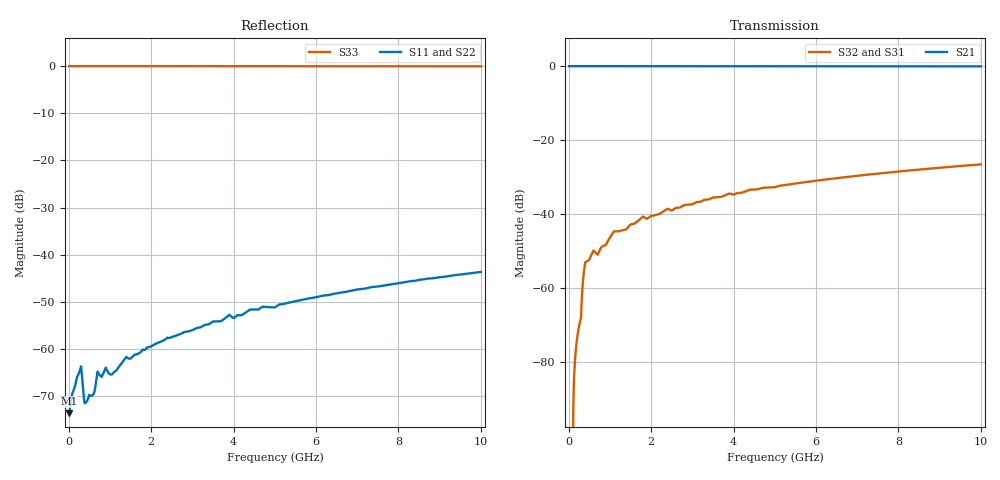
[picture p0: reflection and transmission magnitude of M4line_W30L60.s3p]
! Created Fri Sep 09 14:20:34 2011
# hz S ma R 50
! 3 Port Network Data from SP1.SP block
! freq  magS11  angS11  magS12  angS12  magS13  angS13
!  magS21  angS21
!  magS22  angS22  magS23  angS23
!  magS31  angS31  magS32  angS32
!  magS33  angS33
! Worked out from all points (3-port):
!   1000 points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, 10 MHz to 10 GHz, reference 50 ohm
!   strongest paths, dB at 10 MHz, 2.51 GHz, 5.01 GHz, 7.51 GHz, 10 GHz:
!     S21: 0.0, 0.0, 0.0, 0.0, -0.1
!     S32: -, -39.0, -32.7, -29.1, -26.6
!     S31: -, -39.0, -32.7, -29.1, -26.6
!   lowest |S11| = -73.7 dB at 10 MHz (marker M1), VSWR 1.00, Z = 50 + j0.00283 ohm
!   |S11| at or under -10 dB: start of sweep to end of sweep
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1e7  0.0002073 7.8  0.9998 -0.0  0 0.0
     0.9998 -0.0  0.0002073 7.8  0 0.0
     0 0.0  0 0.0  1 0.0
1.6e8  0.0004155 56.5  0.9998 -0.0  0.00012 90.0
       0.9998 -0.0  0.0004155 56.5  0.00012 90.0
       0.00012 90.0  0.00012 90.0  1 -0.0
2.8e8  0.0006085 66.7  0.9998 -0.1  0.00036 90.0
       0.9998 -0.1  0.0006085 66.7  0.00036 90.0
       0.00036 90.0  0.00036 90.0  1 -0.0
3.7e8  0.0002977 29.4  0.9997 -0.1  0.00166 89.9
       0.9997 -0.1  0.0002977 29.4  0.00166 89.9
       0.00166 89.9  0.00166 89.9  1 -0.2
4.2e8  0.0002711 -0.9  0.9997 -0.1  0.00224 89.8
       0.9997 -0.1  0.0002711 -0.9  0.00224 89.8
       0.00224 89.8  0.00224 89.8  1 -0.3
7.2e8  0.0005547 46.3  0.9996 -0.2  0.00296 89.7
       0.9996 -0.2  0.0005547 46.3  0.00296 89.7
       0.00296 89.7  0.00296 89.7  1 -0.3
1.09e9  0.0005604 -7.4  0.9994 -0.3  0.0057 89.5
        0.9994 -0.3  0.0005604 -7.4  0.0057 89.5
        0.0057 89.5  0.0057 89.5  1 -0.7
2.38e9  0.001298 -14.2  0.9986 -0.6  0.01155 89.0
        0.9986 -0.6  0.001298 -14.2  0.01155 89.0
        0.01155 89.0  0.01155 89.0  0.9999 -1.3
5.01e9  0.002771 -32.8  0.9971 -1.2  0.0231 88.0
        0.9971 -1.2  0.002771 -32.8  0.0231 88.0
        0.0231 88.0  0.0231 88.0  0.9994 -2.6
1e10  0.006549 -58.4  0.994 -2.4  0.04682 85.8
      0.994 -2.4  0.006549 -58.4  0.04682 85.8
      0.04682 85.8  0.04682 85.8  0.9976 -5.4
